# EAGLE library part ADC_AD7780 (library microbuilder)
AD7780 - Low-Power 24-Bit Signma-Delta ADC Converter with 128x PGA For use with load cells TSSOP16 = 5.0x4.4mm package - Digikey: AD7780BRUZ-ND SOIC14 = 8.70x3.9mm package - Digikey: AD7780BRZ-ND
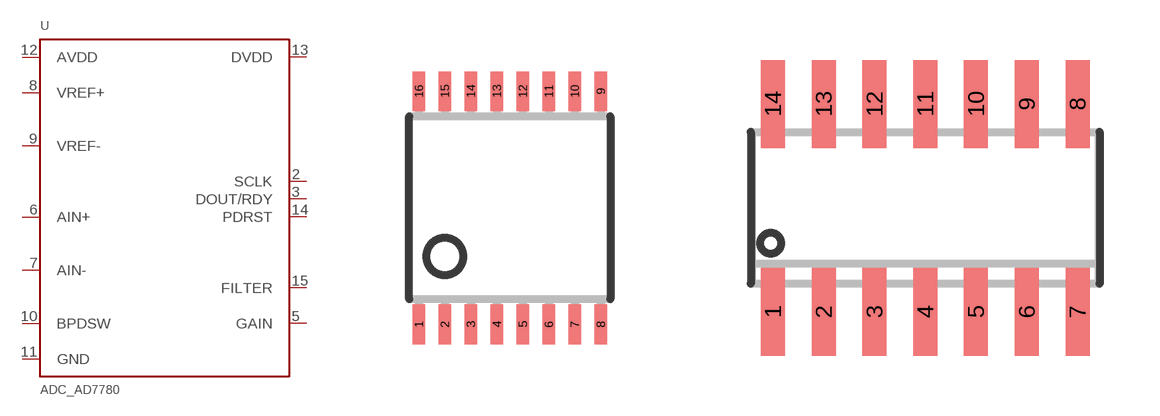
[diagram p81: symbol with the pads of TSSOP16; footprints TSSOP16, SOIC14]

Designator prefix U

## ADC_AD7780  [TSSOP16]
2  SCLK
3  DOUT/RDY
5  GAIN
6  AIN+
7  AIN-
8  VREF+
9  VREF-
10  BPDSW
11  GND
12  AVDD
13  DVDD
14  PDRST
15  FILTER

## ADC_AD7780SOIC  [SOIC14]
1  SCLK
2  DOUT/RDY
4  GAIN
5  AIN+
6  AIN-
7  VREF+
8  VREF-
9  BPDSW
10  GND
11  AVDD
12  DVDD
13  PDRST
14  FILTER

## Footprint TSSOP16 (pad centres in mm)
Thin Shrink Small Outline Plastic 16
smd 0.305 x 0.991: 1 -2.275,-2.918; 2 -1.625,-2.918; 3 -0.975,-2.918; 4 -0.325,-2.918; 5 0.325,-2.918; 6 0.975,-2.918; 7 1.625,-2.918; 8 2.275,-2.918; 9 2.275,2.918; 10 1.625,2.918; 11 0.975,2.918; 12 0.325,2.918; 13 -0.325,2.918; 14 -0.975,2.918; 15 -1.625,2.918; 16 -2.275,2.918

## Footprint SOIC14 (pad centres in mm)
smd 0.6 x 2.2: 1 -3.81,-2.6; 2 -2.54,-2.6; 3 -1.27,-2.6; 4 0,-2.6; 5 1.27,-2.6; 6 2.54,-2.6; 7 3.81,-2.6; 8 3.81,2.6; 9 2.54,2.6; 10 1.27,2.6; 11 0,2.6; 12 -1.27,2.6; 13 -2.54,2.6; 14 -3.81,2.6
